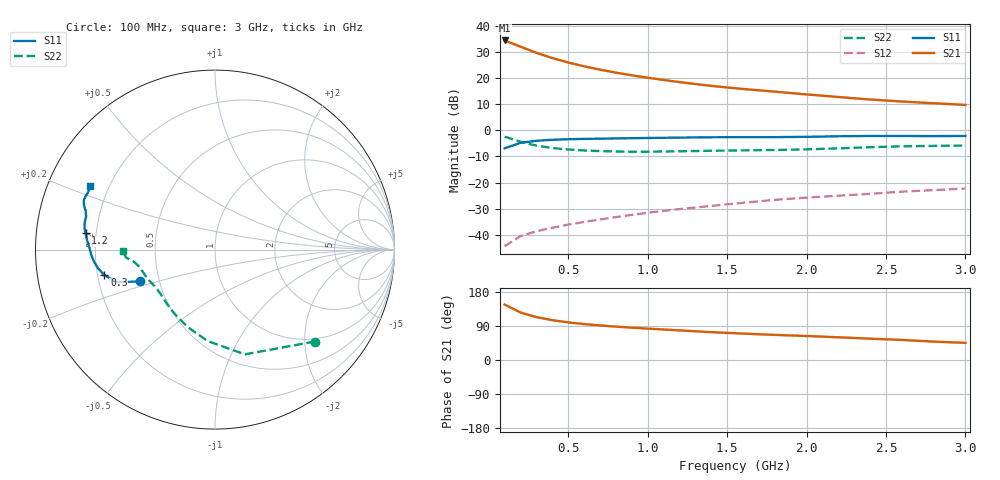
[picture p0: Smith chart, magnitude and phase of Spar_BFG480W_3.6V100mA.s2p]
! Filename: 3_6100BFG480.001
! Title: BFG480W
! Bias: Vce=3.6V; Ic=100mA
! Company: NXP Semiconductors NL
! User: Quality&Reliability T&D
! Measure time: 10 Nov 1999 / 12:01:00
#  MHz  S  MA  R 50
! Freq  S11  S21  S12  S22  :
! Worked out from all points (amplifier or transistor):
!   20 points, 100 MHz to 3 GHz, reference 50 ohm
!   highest |S21| = 34.4 dB at 100 MHz (marker M1)
!   |S21| within 3 dB of that: start of sweep to 226.5 MHz
!   unconditionally stable (mu >= 1): 700.8 MHz to end of sweep
!   at 400 MHz: K = 0.82, MSG = 32.5 dB, |S12| = -37.3 dB
!   at 1.2 GHz: K = 1.08, MAG = 22.6 dB, |S12| = -30.1 dB
!   at 3 GHz: K = 1.05, MAG = 14.6 dB, |S12| = -22.2 dB
!   S11 on the Smith chart (normalised r, x): 100 MHz: 0.39, -0.17; 300 MHz: 0.23, -0.11; 1.2 GHz: 0.16, +0.06; 3 GHz: 0.13, +0.24
100  0.4525 -156.9  52.39 146.4  0.006093 69.5  0.7567 -42.6
200  0.5772 -161.7  39.84 125.3  0.009498 60.6  0.6069 -74.1
300  0.632 -167.0  30.42 113.1  0.01174 59.8  0.511 -94.6
400  0.6598 -170.9  24.14 105.1  0.01369 61.5  0.4592 -108.8
500  0.6758 -174.0  19.87 99.3  0.01571 63.6  0.4303 -119.0
600  0.6863 -176.5  16.77 94.8  0.01769 65.6  0.4129 -126.6
700  0.6936 -178.7  14.49 91.2  0.01975 67.8  0.4014 -132.5
800  0.6999 179.3  12.71 88.0  0.02194 69.3  0.3943 -137.4
900  0.7075 177.4  11.29 85.4  0.02415 71.2  0.3907 -141.6
1000  0.7146 175.7  10.15 82.9  0.02657 72.1  0.3905 -145.4
1200  0.7273 172.8  8.378 78.1  0.03125 73.6  0.3974 -151.4
1400  0.7369 170.5  7.091 73.5  0.03585 74.5  0.4076 -155.9
1600  0.7416 168.2  6.185 69.7  0.04116 75.2  0.4138 -159.4
1800  0.7413 165.6  5.498 66.3  0.04688 75.7  0.4213 -163.0
2000  0.7517 163.4  4.867 63.4  0.05174 76.3  0.4329 -167.3
2200  0.7705 161.3  4.343 59.9  0.05619 76.1  0.4523 -170.9
2400  0.7808 159.6  3.891 56.3  0.06103 75.5  0.4764 -173.2
2600  0.7801 157.9  3.558 53.0  0.06724 74.9  0.4953 -174.7
2800  0.7756 155.6  3.299 48.6  0.07197 73.4  0.5042 -176.5
3000  0.7804 153.0  3.064 45.2  0.07732 72.6  0.5119 -179.3
